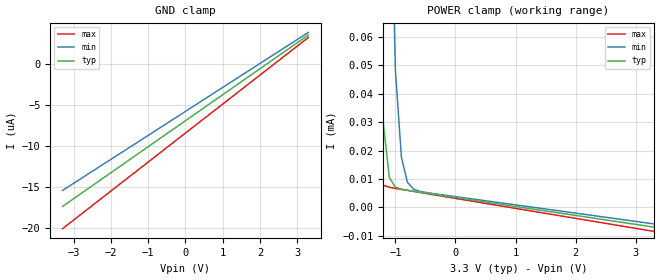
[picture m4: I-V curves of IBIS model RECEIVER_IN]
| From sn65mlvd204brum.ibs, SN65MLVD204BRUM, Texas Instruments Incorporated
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[Model]   RECEIVER_IN
Model_type   Input
Vinl = 1.15V
Vinh = 1.35V
|		 typ	 min	 max
C_comp 6.28152e-12	6.09766e-12	6.45912e-12
[Temperature Range]		 27.0	 125.0	 -40.0
[Voltage range]		 3.3	 3.0	 3.6
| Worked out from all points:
|   POWER clamp passes 1 mA (typ) near -1.46 V on its own axis
[GND_clamp]
|   Voltage   I(typ)   I(min)   I(max)
-3.3V     -17.37uA   -15.43uA   -20.07uA
-200mV    -7.58uA    -6.405uA   -9.157uA
200mV     -6.317uA   -5.231uA   -7.748uA
3.3V      3.475uA    3.789uA    3.17uA
[Power_clamp]
| Note that the[POWER_clamp]voltage table is referenced to Vcc
| and is calculated using Vtable=Vcc - Vmeasured.
|   Voltage   I(typ)   I(min)   I(max)
-1.9V     13.59mA    17.08mA    11.28mA
-1.5V     1.39mA     4.039mA    318.7uA
-1.4V     443.3uA    2.119mA    53.44uA
-1.3V     117.8uA    952.5uA    12.19uA
-1.2V     29.28uA    377.8uA    7.769uA
-1.1V     10.45uA    138.6uA    7.075uA
-1V       7.144uA    48.14uA    6.694uA
-900mV    6.391uA    17.62uA    6.34uA
-800mV    6.012uA    8.845uA    5.987uA
-700mV    5.687uA    6.463uA    5.635uA
-400mV    4.738uA    4.959uA    4.579uA
3.3V      -6.948uA   -5.818uA   -8.452uA
